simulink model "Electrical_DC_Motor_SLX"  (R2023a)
settings: Solver=ode23s  StartTime=0.0  StopTime=10.0  MaxStep=0.001  RelTol=1e-3
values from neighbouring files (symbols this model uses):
  b_7 = 0.1*Nm/(rad/sec)    (= 0.1)    [Electrical_DC_Motor_EQN.m]    (also in Electrical_DC_Motor_SLX_m.m; Car_Dumper_EQN.m = 2; Car_Dumper_SLX_m.m = 2; Electrical_DC_Motor_Pump_and_Load_EQN.m)
  I_2_0 = 0*A    (= 0)    [Electrical_DC_Motor_SLX_m.m]    (also in Electric_Circuit_02_SLX_m.m; Electric_Circuit_03_SLX_m.m; Electric_Circuit_06_SLX_m.m; Electric_Circuit_08_SLX_m.m)
  J_6 = 0.01*kg*m^2    (= 0.01)    [Electrical_DC_Motor_EQN.m]    (also in Electrical_DC_Motor_SLX_m.m; Electrical_DC_Motor_Pump_and_Load_EQN.m; Electrical_DC_Motor_Pump_and_Load_SLX_m.m; Electrical_DC_Motor_and_Pump_EQN.m)
  K = 1    [Electrical_DC_Motor_EQN.m]    (also in Electrical_DC_Motor_SLX_m.m; SI_Units.m)
  L_2 = 0.002*H    (= 0.002)    [Electrical_DC_Motor_EQN.m]    (also in Electrical_DC_Motor_SLX_m.m; Electric_Circuit_02_EQN.m; Electric_Circuit_02_SLX_m.m; Electric_Circuit_03_EQN.m)
  R_3 = 100*Ohm    (= 100)    [Electrical_DC_Motor_EQN.m]    (also in Electrical_DC_Motor_SLX_m.m; Electric_Circuit_01_EQN.m; Electric_Circuit_01_SLX_m.m; Electric_Circuit_02_EQN.m)
  T_8_0 = 0*Nm    (= 0)    [Electrical_DC_Motor_SLX_m.m]    (also in Rotational_Inertias_and_Dumper_SLX_m.m)
  Ts = Tfin/Nr_Ts_Points    (= 0.00027272)    [Electrical_DC_Motor_SLX_m.m]    (also in BIG_EC_Simscape_SLX_m.m = 0.0003; Car_Dumper_SLX_m.m = 0.0022779; Electric_Circuit_01_SLX_m.m = 0.005; Electric_Circuit_02_SLX_m.m = 0.000480145)
  V_1_0 = 10*V    (= 10)    [Electrical_DC_Motor_SLX_m.m]    (also in BIG_EC_Simscape_SLX_m.m; Electric_Circuit_02_SLX_m.m; Electric_Circuit_03_SLX_m.m; Electric_Circuit_04_SLX_m.m)
  w_6_0 = 0*rad/sec    (= 0)    [Electrical_DC_Motor_SLX_m.m]    (also in Electrical_DC_Motor_Pump_and_Load_SLX_m.m; Electrical_DC_Motor_and_Pump_SLX_m.m)

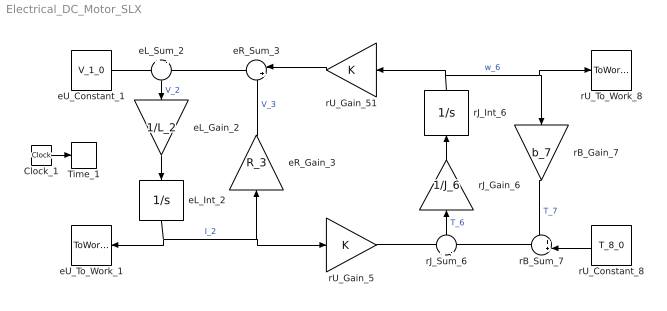
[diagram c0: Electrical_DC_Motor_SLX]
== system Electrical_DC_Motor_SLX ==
  Clock_1 : Clock
  Time_1 : ToWorkspace  VariableName=t  SaveFormat=Timeseries  SampleTime=Ts
  eL_Gain_2 : Gain  Gain=1/L_2  Multiplication=Matrix(K*u)
  eL_Int_2 : Integrator  InitialCondition=I_2_0
  eL_Sum_2 : Sum  Inputs=+|-
  eR_Gain_3 : Gain  Gain=R_3  Multiplication=Matrix(K*u)
  eR_Sum_3 : Sum  Inputs=|++
  eU_Constant_1 : Constant  Value=V_1_0
  eU_To_Work_1 : ToWorkspace  VariableName=I_1_0  SaveFormat=Timeseries  SampleTime=Ts
  rB_Gain_7 : Gain  Gain=b_7  Multiplication=Matrix(K*u)
  rB_Sum_7 : Sum  Inputs=++|
  rJ_Gain_6 : Gain  Gain=1/J_6  Multiplication=Matrix(K*u)
  rJ_Int_6 : Integrator  InitialCondition=w_6_0
  rJ_Sum_6 : Sum  Inputs=+|-
  rU_Constant_8 : Constant  Value=T_8_0
  rU_Gain_5 : Gain  Gain=K  Multiplication=Matrix(K*u)
  rU_Gain_51 : Gain  Gain=K  Multiplication=Matrix(K*u)
  rU_To_Work_8 : ToWorkspace  VariableName=w_8_0  SaveFormat=Timeseries  SampleTime=Ts
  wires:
  eU_Constant_1/1 -> eL_Sum_2/1
  eR_Sum_3/1 -> eL_Sum_2/2
  eL_Int_2/1 -> eU_To_Work_1/1, eR_Gain_3/1, rU_Gain_5/1  "I_2"
  eL_Sum_2/1 -> eL_Gain_2/1  "V_2"
  eL_Gain_2/1 -> eL_Int_2/1
  rU_Gain_51/1 -> eR_Sum_3/1
  eR_Gain_3/1 -> eR_Sum_3/2  "V_3"
  rU_Gain_5/1 -> rJ_Sum_6/1
  rJ_Int_6/1 -> rU_Gain_51/1, rU_To_Work_8/1, rB_Gain_7/1  "w_6"
  rB_Sum_7/1 -> rJ_Sum_6/2
  rJ_Sum_6/1 -> rJ_Gain_6/1  "T_6"
  rJ_Gain_6/1 -> rJ_Int_6/1
  rU_Constant_8/1 -> rB_Sum_7/2
  rB_Gain_7/1 -> rB_Sum_7/1  "T_7"
  Clock_1/1 -> Time_1/1
